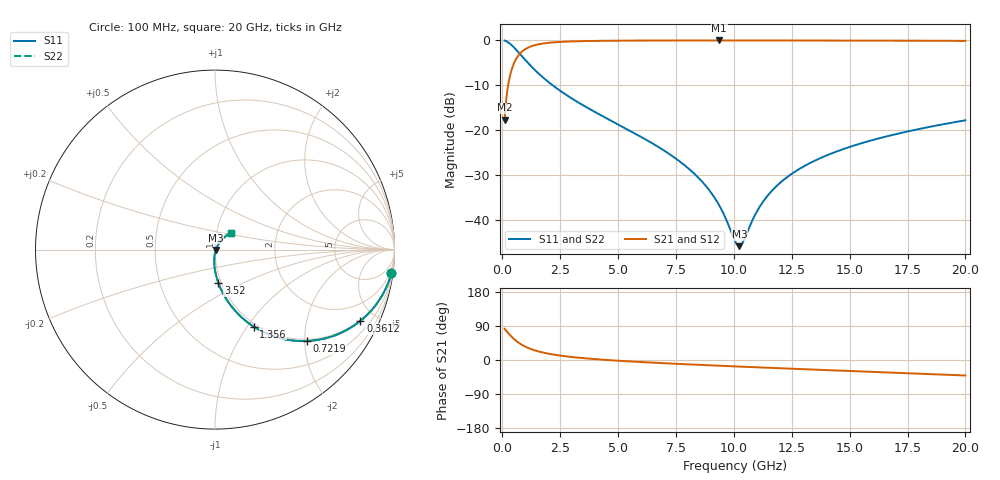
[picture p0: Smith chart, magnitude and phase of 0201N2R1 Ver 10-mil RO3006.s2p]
# GHz S MA R 50
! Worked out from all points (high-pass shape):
!   1601 points, 100 MHz to 20 GHz, reference 50 ohm
!   highest |S21| = -0.05 dB at 9.366 GHz (marker M1); lowest = -17.7 dB at 100 MHz (marker M2)
!   |S21| within 3 dB of the highest: 749.7 MHz to end of sweep
!   lowest |S11| = -45.8 dB at 10.24 GHz (marker M3), VSWR 1.01, Z = 50.5 - j0.153 ohm
!   |S11| at or under -10 dB: 2.17 GHz to end of sweep
!   |S22| runs from -45.8 to -0.1 dB; largest |S21 - S12| = 0
!   S11 on the Smith chart (normalised r, x): 100 MHz: 1, -15; 361.2 MHz: 0.96, -4.10; 721.9 MHz: 0.96, -2.04; 1.356 GHz: 0.96, -1.07; 3.52 GHz: 0.97, -0.37; 20 GHz: 1.17, +0.22
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0.1  0.9914 -7.7  0.1309 82.3  0.1309 82.3  0.9914 -7.7
0.2616875  0.9449 -19.5  0.3265 70.4  0.3265 70.4  0.9449 -19.5
0.3611875  0.9021 -26.1  0.4305 63.8  0.4305 63.8  0.9021 -26.1
0.522875  0.8217 -35.5  0.5685 54.4  0.5685 54.4  0.8217 -35.5
0.721875  0.7215 -44.9  0.6906 44.9  0.6906 44.9  0.7215 -44.9
1.020375  0.5915 -55.3  0.8041 34.5  0.8041 34.5  0.5915 -55.3
1.356188  0.4805 -63.3  0.8745 26.4  0.8745 26.4  0.4805 -63.3
2.13975  0.3206 -74.4  0.9442 15.0  0.9442 15.0  0.3206 -74.4
3.420812  0.1937 -83.6  0.9775 5.3  0.9775 5.3  0.1937 -83.6
3.520313  0.1871 -84.2  0.9787 4.8  0.9787 4.8  0.1871 -84.2
6.741625  0.06503 -93.9  0.9933 -7.8  0.9933 -7.8  0.06503 -93.9
8.333625  0.03206 -93.9  0.9945 -12.4  0.9945 -12.4  0.03206 -93.9
9.365937  0.01462 -85.3  0.9947 -15.1  0.9947 -15.1  0.01462 -85.3
10.05  0.005837 -46.1  0.9946 -16.9  0.9946 -16.9  0.005837 -46.1
10.23656  0.00513 -17.2  0.9946 -17.4  0.9946 -17.4  0.00513 -17.2
10.41069  0.005806 9.4  0.9946 -17.8  0.9946 -17.8  0.005806 9.4
11.045  0.01311 46.8  0.9944 -19.4  0.9944 -19.4  0.01311 46.8
11.55494  0.01999 53.7  0.9941 -20.7  0.9941 -20.7  0.01999 53.7
12.3385  0.03056 57.0  0.9937 -22.6  0.9937 -22.6  0.03056 57.0
13.37081  0.04417 57.4  0.993 -25.1  0.993 -25.1  0.04417 57.4
16.69162  0.08647 52.8  0.9896 -33.1  0.9896 -33.1  0.08647 52.8
20  0.1288 46.1  0.9843 -40.9  0.9843 -40.9  0.1288 46.1
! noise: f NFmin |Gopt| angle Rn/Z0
0.1  0.0009605  0.9561  0.6222  0.004926
2.301  0.005358  0.8259  4.264  0.006461
4.515  0.008286  0.7843  7.943  0.007855
6.729  0.01081  0.7577  11.62  0.008938
8.943  0.01312  0.7383  15.27  0.009855
11.14  0.01527  0.7233  18.87  0.01066
13.36  0.01735  0.7112  22.46  0.0114
15.57  0.01937  0.7015  26.01  0.01209
17.79  0.02135  0.6937  29.51  0.01274
20  0.0233  0.6873  32.97  0.01335
